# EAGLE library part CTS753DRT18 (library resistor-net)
Network Resistor CTS 753 Series Leadless Surface Mount Source: http://www.ctscorp.com/components/Datasheets/753.pdf Distributor: Digi Key
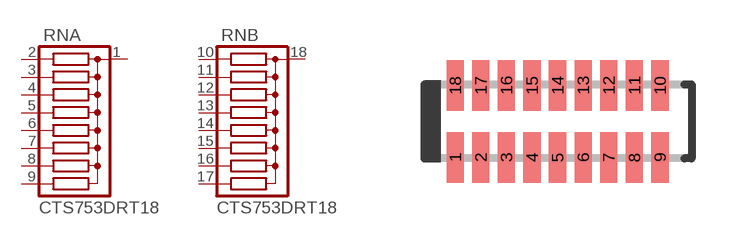
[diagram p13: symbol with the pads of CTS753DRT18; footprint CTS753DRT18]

Designator prefix RN; gates A=RN1X8 B=RN1X8

## CTS753DRT18 (OC_FARNELL: unknown; OC_NEWARK: unknown)  [CTS753DRT18]
1  A:C  pas
2  A:1  pas
3  A:2  pas
4  A:3  pas
5  A:4  pas
6  A:5  pas
7  A:6  pas
8  A:7  pas
9  A:8  pas
10  B:1  pas
11  B:2  pas
12  B:3  pas
13  B:4  pas
14  B:5  pas
15  B:6  pas
16  B:7  pas
17  B:8  pas
18  B:C  pas

## Footprint CTS753DRT18 (pad centres in mm)
Network Resistor Leadless Surface Mount Series 753 Source: http://www.ctscorp.com/components/Datasheets/753.pdf
smd 0.43 x 1.27: 1 -2.56,-0.9; 2 -1.92,-0.9; 3 -1.28,-0.9; 4 -0.64,-0.9; 5 0,-0.9; 6 0.64,-0.9; 7 1.28,-0.9; 8 1.92,-0.9; 9 2.56,-0.9; 10 2.56,0.9; 11 1.92,0.9; 12 1.28,0.9; 13 0.64,0.9; 14 0,0.9; 15 -0.64,0.9; 16 -1.28,0.9; 17 -1.92,0.9; 18 -2.56,0.9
